ORGANIZATION_BLOCK "Hardware Interrupt 3"
TITLE =
VERSION : 0.1


VAR_TEMP
  OB43_EV_CLASS : BYTE ;	//Bits 0-3 = 1 (Coming event), Bits 4-7 = 1 (Event class 1)
  OB43_STRT_INF : BYTE ;	//16#41/42/43/44 (Interrupt 1/2/3/4)
  OB43_PRIORITY : BYTE ;	//19 (Priority of 1 is lowest)
  OB43_OB_NUMBR : BYTE ;	//43 (Organization block 43, OB43)
  OB43_RESERVED_1 : BYTE ;	//Reserved for system
  OB43_RESERVED_2 : BYTE ;	//Reserved for system
  OB43_MDL_ADDR : WORD ;	//Base address of module initiating interrupt
  OB43_POINT_ADDR : DWORD ;	//Address of interrupt point on module
  OB43_DATE_TIME : DATE_AND_TIME ;	//Date and time OB43 started
END_VAR
BEGIN
END_ORGANIZATION_BLOCK

